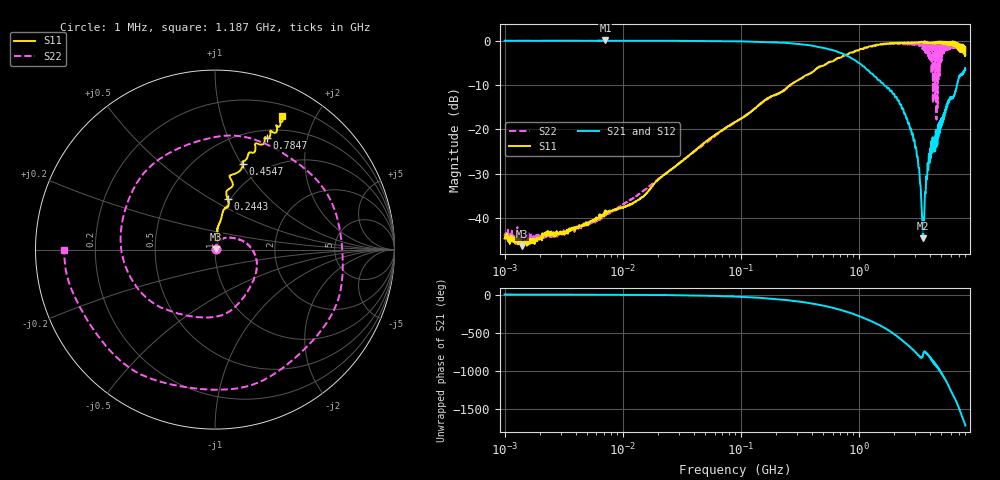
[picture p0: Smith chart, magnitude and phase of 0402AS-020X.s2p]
!s-Parameter Generated by FASTRON Sdn. Bhd.
!FASTRON P/N : 0402AS-020X
!Keysight Technologies: E5071C_MY46733604_B.14.02
!Date: Mon Dec 01 10:32:33 2025
!Version  :Rev00  Mon Dec 01 10:32:33 2025
!Data & Calibration Information:
!Freq  S11:SOLT2(ON)  S21:SOLT2(ON)  S12:SOLT2(ON)  S22:SOLT2(ON)
!PortZ  Port1:50+j0  Port2:50+j0
!When reading reference impedance value at option line is always used.
! Remarks : This data is being provided solely for informational purposes.
# Hz S dB R 50
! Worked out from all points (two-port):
!   1601 points, 1 MHz to 8 GHz, reference 50 ohm
!   highest |S21| = 0.01 dB at 7.138 MHz (marker M1); lowest = -44.5 dB at 3.487 GHz (marker M2)
!   |S21| within 3 dB of the highest: start of sweep to 735.7 MHz
!   lowest |S11| = -46.3 dB at 1.405 MHz (marker M3), VSWR 1.01, Z = 50.5 + j0.181 ohm
!   |S11| at or under -10 dB: start of sweep to 261.4 MHz
!   |S22| runs from -45.8 to -0.1 dB; largest |S21 - S12| = 0.027
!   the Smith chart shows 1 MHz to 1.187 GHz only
!   S11 on the Smith chart (normalised r, x): 1 MHz: 1.01, +0.00; 244.3 MHz: 0.97, +0.60; 454.7 MHz: 0.79, +1.01; 784.7 MHz: 0.59, +1.40; 1.187 GHz: 0.32, +1.57
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1000000  -44.60 18.1  -0.06 -0.3  -0.05 -0.3  -43.50 13.0
1404635  -46.30 21.7  -0.07 -0.5  -0.05 -0.5  -44.70 5.8
4479405  -41.60 45.9  -0.07 -1.4  -0.05 -1.4  -41.80 50.1
7138274  -38.20 52.8  0.01 -2.4  -0.07 -2.2  -38.60 54.0
2.00676e7  -31.30 69.1  -0.07 -6.2  -0.07 -6.1  -31.20 68.8
8.994653e7  -18.30 83.1  -0.17 -27.1  -0.17 -27.1  -18.40 32.6
2.443405e8  -10.70 76.0  -0.54 -72.3  -0.54 -72.3  -10.90 -46.3
4.006501e8  -7.23 75.6  -1.15 -117.0  -1.14 -117.0  -7.09 -133.0
4.547402e8  -5.96 72.2  -1.46 -133.0  -1.46 -133.0  -6.16 -160.0
7.847468e8  -3.26 65.0  -3.39 136.0  -3.38 136.0  -3.13 26.9
1.002268e9  -2.17 62.3  -5.04 79.2  -5.04 79.0  -2.14 -86.0
1.187136e9  -1.60 63.5  -6.62 33.0  -6.63 32.8  -1.51 180.0
1.542898e9  -0.81 70.6  -9.42 -51.4  -9.43 -51.5  -0.86 3.3
1.7949e9  -0.65 76.0  -10.70 -110.0  -10.80 -110.0  -0.80 -119.0
2.082516e9  -0.59 81.9  -12.70 -179.0  -12.70 -179.0  -0.78 98.0
2.266813e9  -0.66 83.7  -14.40 138.0  -14.30 138.0  -0.71 8.7
2.457552e9  -0.66 87.1  -16.40 93.4  -16.40 93.4  -0.65 -84.0
2.809687e9  -0.51 96.0  -21.10 13.2  -21.10 12.9  -0.46 101.0
3.183204e9  -0.41 105.0  -27.60 -72.4  -27.60 -72.7  -0.85 -89.8
3.487237e9  -0.36 112.0  -44.50 -77.2  -44.80 -77.9  -0.64 114.0
3.933151e9  -0.60 121.0  -25.50 -87.7  -25.70 -87.2  -3.23 -89.2
8e9  -1.55 -110.0  -6.54 89.5  -6.57 89.3  -3.08 126.0
